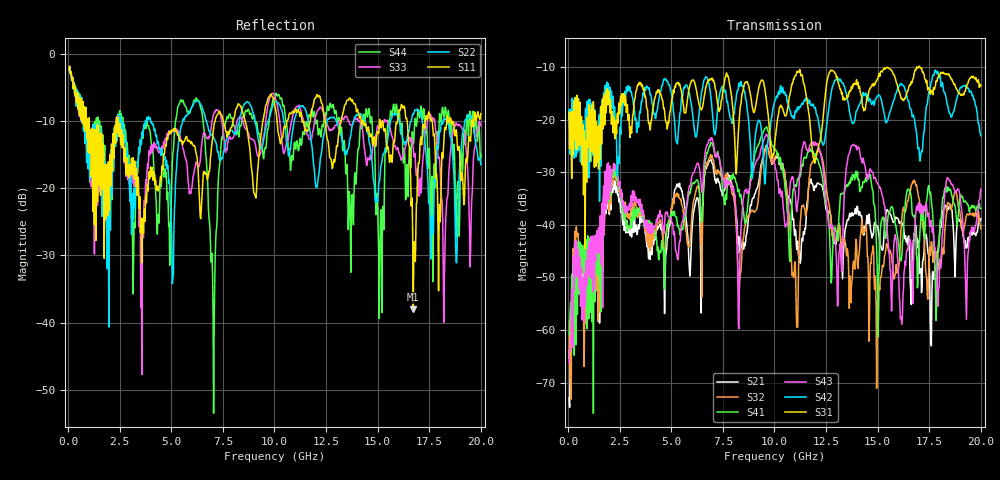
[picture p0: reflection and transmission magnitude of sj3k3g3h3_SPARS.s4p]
! FILE: E:\users\goganessyan\GBX_Backplane\FR408_backplane\1m_OUTBOUND_NEXT\sj3k3g3h3_SPARS.s4p
# MHZ S RI R 50.00
! FREQ  S11  S12  S13  S14
!  S21  S22  S23  S24
!  S31  S32  S33  S34
!  S41  S42  S43  S44
!  REAL  IMAG  REAL  IMAG  REAL  IMAG  REAL  IMAG
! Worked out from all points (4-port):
!   799 points, 50 MHz to 20 GHz, reference 50 ohm
!   strongest paths, dB at 50 MHz, 5.025 GHz, 10.03 GHz, 15.03 GHz, 20 GHz:
!     S31: -18.6, -16.1, -23.9, -12.0, -13.6
!     S42: -18.1, -15.7, -16.4, -15.3, -23.1
!     S43: -66.1, -39.7, -28.7, -32.3, -33.2
!     S41: -60.8, -38.3, -25.6, -61.3, -36.9
!     S32: -65.4, -36.4, -27.1, -60.1, -40.8
!     S21: -72.9, -36.7, -27.5, -41.1, -38.9
!   lowest |S11| = -38.0 dB at 16.73 GHz (marker M1), VSWR 1.03, Z = 50 - j1.26 ohm
!   |S11| at or under -10 dB: 1.027 GHz to 2.332 GHz (1.305 GHz wide, 77.7 % of centre); 2.432 GHz to 7.123 GHz (4.691 GHz wide, 98.2 % of centre); 18.56 GHz to 19.56 GHz (1 GHz wide, 5.25 % of centre)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
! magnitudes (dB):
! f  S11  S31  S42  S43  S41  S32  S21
! 50 MHz  -2.5  -18.6  -18.1  -66.1  -60.8  -65.4  -72.9
! 2.275 GHz  -10.7  -23.6  -19.4  -28.6  -29.3  -30.0  -31.7
! 11.07 GHz  -8.6  -11.1  -18.5  -37.5  -32.5  -59.3  -44.7
! 12.15 GHz  -6.4  -24.7  -20.8  -25.3  -28.4  -25.8  -32.2
! 15 GHz  -11.6  -12.2  -15.4  -32.2  -55.1  -54.5  -40.3
! 16.73 GHz  -38.0  -12.2  -19.1  -48.5  -38.2  -32.0  -43.0
! 20 GHz  -8.9  -13.6  -23.1  -33.2  -36.9  -40.8  -38.9
